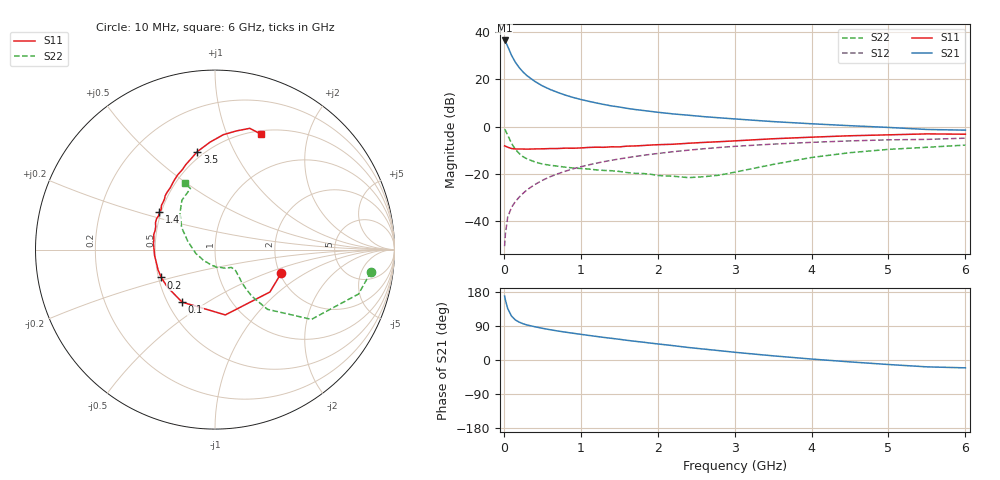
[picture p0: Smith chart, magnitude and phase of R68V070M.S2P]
! SIEMENS Small Signal Semiconductors
! BFR193
! Si NPN RF Bipolar Junction Transistor in SOT23
! VCE = 8 V  IC = 70 mA
! Common Emitter S-Parameters:  May  1996
# GHz  S  MA  R  50
!  f  S11  S21  S12  S22
! GHz  MAG  ANG  MAG  ANG  MAG  ANG  MAG  ANG
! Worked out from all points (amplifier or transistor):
!   36 points, 10 MHz to 6 GHz, reference 50 ohm
!   highest |S21| = 36.4 dB at 10 MHz (marker M1)
!   |S21| within 3 dB of that: start of sweep to 56.71 MHz
!   unconditionally stable (mu >= 1): 374.7 MHz to 2.19 GHz
!   at 250 MHz: K = 0.96, MSG = 25.6 dB, |S12| = -28.2 dB
!   at 1.4 GHz: K = 1.03, MAG = 10.5 dB, |S12| = -14.2 dB
!   at 6 GHz: K = 0.95, MSG = 1.7 dB, |S12| = -4.9 dB
!   S11 on the Smith chart (normalised r, x): 10 MHz: 2.04, -0.63; 100 MHz: 0.59, -0.39; 200 MHz: 0.52, -0.18; 1.4 GHz: 0.49, +0.24; 3.5 GHz: 0.46, +0.73; 6 GHz: 0.54, +1.33
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0.01  0.3918 -19.5  65.87 168.7  0.003 80.5  0.8778 -8.1
0.02  0.3865 -37.7  62.83 158.6  0.0054 73.0  0.8371 -17.2
0.05  0.3684 -81.0  49.45 135.8  0.0123 69.4  0.6632 -35.9
0.1  0.3452 -122.0  31.97 115.9  0.0198 67.6  0.4429 -48.7
0.15  0.3377 -141.4  22.79 105.7  0.0263 68.2  0.3306 -51.7
0.2  0.3375 -152.6  17.59 99.9  0.0325 70.7  0.2706 -51.6
0.25  0.3367 -160.6  14.21 95.7  0.0391 72.7  0.2315 -50.6
0.3  0.3347 -165.4  11.94 92.5  0.0462 73.6  0.2096 -49.2
0.4  0.3383 -174.4  9.072 87.9  0.0596 74.2  0.1807 -47.1
0.5  0.34 179.2  7.269 83.7  0.0734 73.9  0.1627 -45.6
0.6  0.3443 174.5  6.103 80.0  0.0874 73.1  0.1532 -45.6
0.8  0.3518 166.2  4.622 73.5  0.1147 71.1  0.1394 -47.2
0.9  0.35 162.3  4.131 70.6  0.1287 70.2  0.1339 -47.7
1.1  0.3637 155.8  3.434 65.0  0.1553 67.7  0.1275 -53.0
1.4  0.3749 145.7  2.736 57.2  0.1949 63.6  0.1173 -61.1
1.7  0.3909 137.9  2.305 49.5  0.2337 59.3  0.1032 -72.8
2.2  0.4249 126.0  1.856 37.9  0.2955 51.7  0.0898 -102.5
2.8  0.4808 112.3  1.537 24.7  0.3631 42.5  0.0945 -155.3
3.5  0.5548 100.2  1.277 11.0  0.4276 31.4  0.1595 162.6
4.5  0.6417 85.9  1.046 -5.0  0.5001 17.5  0.2821 133.8
5.5  0.7029 74.0  0.871 -18.1  0.5379 3.9  0.3668 111.9
6  0.6921 68.2  0.843 -20.7  0.5712 0.1  0.4075 114.2
